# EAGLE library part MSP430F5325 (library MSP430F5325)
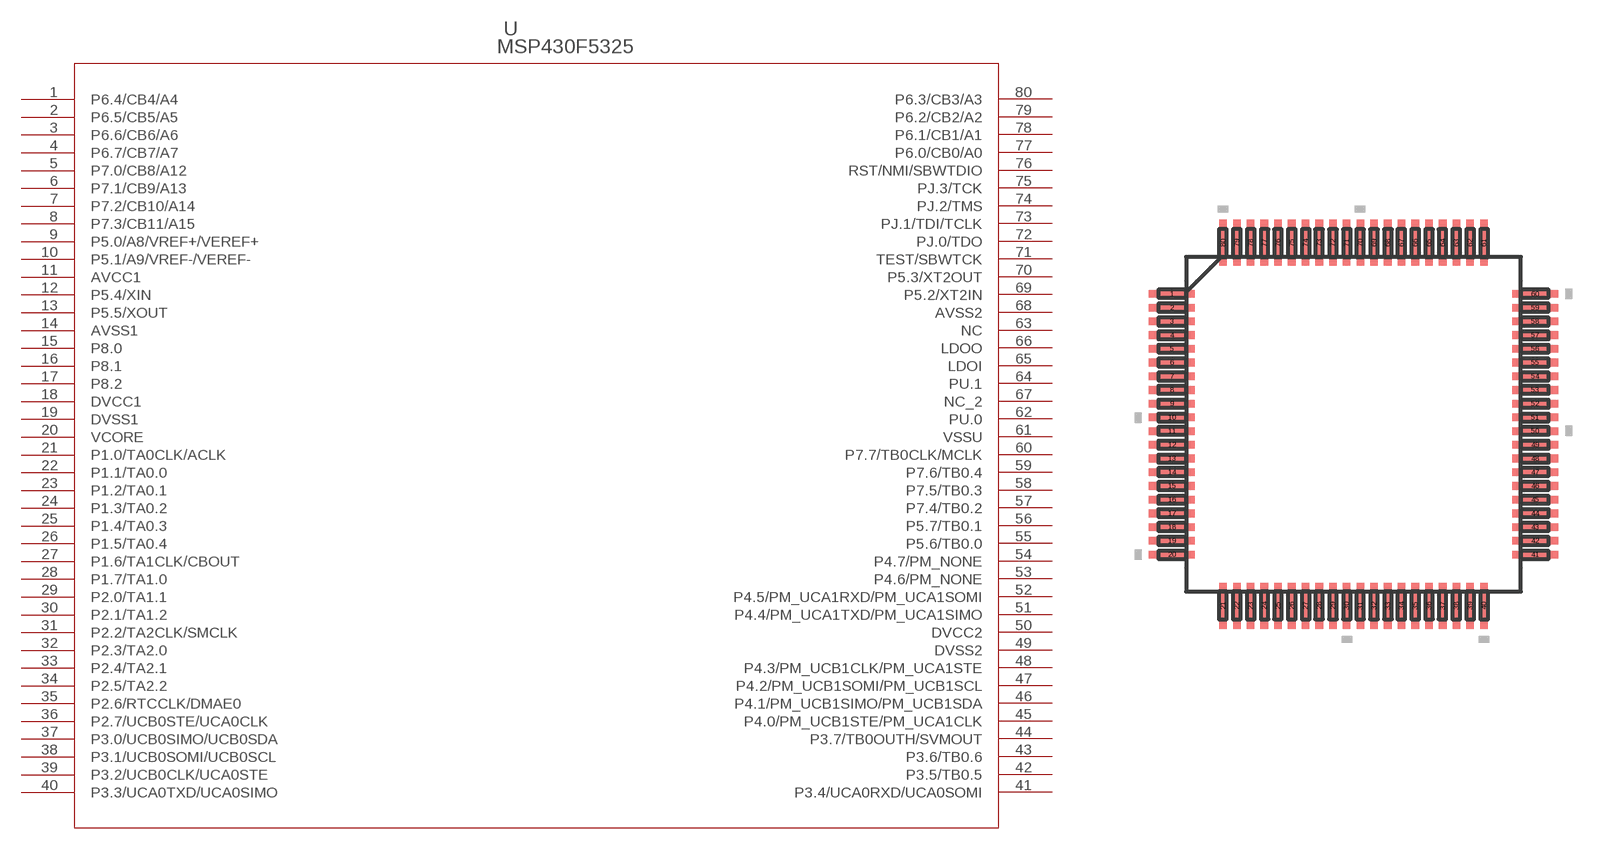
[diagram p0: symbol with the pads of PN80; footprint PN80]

Designator prefix -

## MSP430F5325  [PN80]
1  P6.4/CB4/A4
2  P6.5/CB5/A5
3  P6.6/CB6/A6
4  P6.7/CB7/A7
5  P7.0/CB8/A12
6  P7.1/CB9/A13
7  P7.2/CB10/A14
8  P7.3/CB11/A15
9  P5.0/A8/VREF+/VEREF+
10  P5.1/A9/VREF-/VEREF-
11  AVCC1  pwr
12  P5.4/XIN
13  P5.5/XOUT
14  AVSS1  pwr
15  P8.0
16  P8.1
17  P8.2
18  DVCC1  pwr
19  DVSS1  pwr
20  VCORE  pwr
21  P1.0/TA0CLK/ACLK
22  P1.1/TA0.0
23  P1.2/TA0.1
24  P1.3/TA0.2
25  P1.4/TA0.3
26  P1.5/TA0.4
27  P1.6/TA1CLK/CBOUT
28  P1.7/TA1.0
29  P2.0/TA1.1
30  P2.1/TA1.2
31  P2.2/TA2CLK/SMCLK
32  P2.3/TA2.0
33  P2.4/TA2.1
34  P2.5/TA2.2
35  P2.6/RTCCLK/DMAE0
36  P2.7/UCB0STE/UCA0CLK
37  P3.0/UCB0SIMO/UCB0SDA
38  P3.1/UCB0SOMI/UCB0SCL
39  P3.2/UCB0CLK/UCA0STE
40  P3.3/UCA0TXD/UCA0SIMO
41  P3.4/UCA0RXD/UCA0SOMI
42  P3.5/TB0.5
43  P3.6/TB0.6
44  P3.7/TB0OUTH/SVMOUT
45  P4.0/PM_UCB1STE/PM_UCA1CLK
46  P4.1/PM_UCB1SIMO/PM_UCB1SDA
47  P4.2/PM_UCB1SOMI/PM_UCB1SCL
48  P4.3/PM_UCB1CLK/PM_UCA1STE
49  DVSS2  pwr
50  DVCC2  pwr
51  P4.4/PM_UCA1TXD/PM_UCA1SIMO
52  P4.5/PM_UCA1RXD/PM_UCA1SOMI
53  P4.6/PM_NONE
54  P4.7/PM_NONE
55  P5.6/TB0.0
56  P5.7/TB0.1
57  P7.4/TB0.2
58  P7.5/TB0.3
59  P7.6/TB0.4
60  P7.7/TB0CLK/MCLK
61  VSSU  pwr
62  PU.0
63  NC  pas
64  PU.1
65  LDOI  in
66  LDOO  out
67  NC_2  pas
68  AVSS2  pwr
69  P5.2/XT2IN
70  P5.3/XT2OUT
71  TEST/SBWTCK
72  PJ.0/TDO
73  PJ.1/TDI/TCLK
74  PJ.2/TMS
75  PJ.3/TCK
76  RST/NMI/SBWTDIO
77  P6.0/CB0/A0
78  P6.1/CB1/A1
79  P6.2/CB2/A2
80  P6.3/CB3/A3

## Footprint PN80 (pad centres in mm)
smd 1.676 x 0.279: 1 -6.617,4.75; 2 -6.617,4.25; 3 -6.617,3.75; 4 -6.617,3.25; 5 -6.617,2.75; 6 -6.617,2.25; 7 -6.617,1.75; 8 -6.617,1.25; 9 -6.617,0.75; 10 -6.617,0.25; 11 -6.617,-0.25; 12 -6.617,-0.75; 13 -6.617,-1.25; 14 -6.617,-1.75; 15 -6.617,-2.25; 16 -6.617,-2.75; 17 -6.617,-3.25; 18 -6.617,-3.75; 19 -6.617,-4.25; 20 -6.617,-4.75; 41 6.617,-4.75; 42 6.617,-4.25; 43 6.617,-3.75; 44 6.617,-3.25; 45 6.617,-2.75; 46 6.617,-2.25; 47 6.617,-1.75; 48 6.617,-1.25; 49 6.617,-0.75; 50 6.617,-0.25; 51 6.617,0.25; 52 6.617,0.75; 53 6.617,1.25; 54 6.617,1.75; 55 6.617,2.25; 56 6.617,2.75; 57 6.617,3.25; 58 6.617,3.75; 59 6.617,4.25; 60 6.617,4.75
smd 0.279 x 1.676: 21 -4.75,-6.617; 22 -4.25,-6.617; 23 -3.75,-6.617; 24 -3.25,-6.617; 25 -2.75,-6.617; 26 -2.25,-6.617; 27 -1.75,-6.617; 28 -1.25,-6.617; 29 -0.75,-6.617; 30 -0.25,-6.617; 31 0.25,-6.617; 32 0.75,-6.617; 33 1.25,-6.617; 34 1.75,-6.617; 35 2.25,-6.617; 36 2.75,-6.617; 37 3.25,-6.617; 38 3.75,-6.617; 39 4.25,-6.617; 40 4.75,-6.617; 61 4.75,6.617; 62 4.25,6.617; 63 3.75,6.617; 64 3.25,6.617; 65 2.75,6.617; 66 2.25,6.617; 67 1.75,6.617; 68 1.25,6.617; 69 0.75,6.617; 70 0.25,6.617; 71 -0.25,6.617; 72 -0.75,6.617; 73 -1.25,6.617; 74 -1.75,6.617; 75 -2.25,6.617; 76 -2.75,6.617; 77 -3.25,6.617; 78 -3.75,6.617; 79 -4.25,6.617; 80 -4.75,6.617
